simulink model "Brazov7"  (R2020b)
settings: Solver=VariableStepAuto  StartTime=0.0  StopTime=10.0  RelTol=1e-3
model workspace: external: MAT-File (data not in the file)
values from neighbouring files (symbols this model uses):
  q1 = 0    [angles.m]
  q2 = 90    [angles.m]
  q3 = 90    [angles.m]
  q4 = 0    [angles.m]
  q5 = 0    [angles.m]
undefined symbols (not defined in the file or in its folder): deg, kg, m, mm, N, s, smiData, X, Y, Z
libraries: sm_lib x30, nesl_utility x6

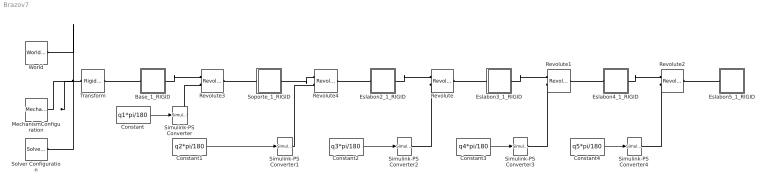
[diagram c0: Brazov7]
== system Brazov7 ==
  Base_1_RIGID : Subsystem
  Constant : Constant  Value=q1*pi/180
  Constant1 : Constant  Value=q2*pi/180
  Constant2 : Constant  Value=q3*pi/180
  Constant3 : Constant  Value=q4*pi/180
  Constant4 : Constant  Value=q5*pi/180
  Eslabon2_1_RIGID : Subsystem
  Eslabon3_1_RIGID : Subsystem
  Eslabon4_1_RIGID : Subsystem
  Eslabon5_1_RIGID : Subsystem
  MechanismConfiguration : sm_lib/Utilities/Mechanism Configuration  UniformGravity=Constant  GravityVector=[0 -9.80665 0]  GravityVectorUnits=m/s^2  GravityUnits=m/s^2  LinearizationDelta=0.001  JointModeTransitionNonlinearIterations=2
  Revolute : sm_lib/Joints/Revolute Joint  JointMode=Normal  SenseConstraintForce=off  SenseConstraintForceX=off  SenseConstraintForceY=off  SenseConstraintForceZ=off  SenseConstraintTorque=off  SenseConstraintTorqueX=off  SenseConstraintTorqueY=off  SenseConstraintTorqueZ=off  SenseTotalForce=off  SenseTotalForceX=off  SenseTotalForceY=off  SenseTotalForceZ=off  SenseTotalTorque=off  SenseTotalTorqueX=off  SenseTotalTorqueY=off  SenseTotalTorqueZ=off  CompositeWrenchDir=FollowerOnBase  CompositeWrenchFrame=BaseFrame  EquilibriumPosition=0  EquilibriumPositionUnits=deg  SpringStiffness=0  SpringStiffnessUnits=N*m/deg  DampingCoefficient=0  DampingCoefficientUnits=N*m/(deg/s)  TorqueActuationMode=ComputedTorque  MotionActuationMode=InputMotion  SensePosition=off  SenseVelocity=off  SenseAcceleration=off  SenseTorqueForce=off  SenseLowerLimitTorqueForce=off  SenseUpperLimitTorqueForce=off  LowerLimitSpecify=off  LowerLimitBound=-90  LowerLimitBoundUnits=deg  LowerLimitStiffness=1e4  LowerLimitStiffnessUnits=N*m/deg  LowerLimitDamping=10  LowerLimitDampingUnits=N*m/(deg/s)  LowerLimitTransitionRegionWidth=0.1  LowerLimitTransitionRegionWidthUnits=deg  UpperLimitSpecify=off  UpperLimitBound=90  UpperLimitBoundUnits=deg  UpperLimitStiffness=1e4  UpperLimitStiffnessUnits=N*m/deg  UpperLimitDamping=10  UpperLimitDampingUnits=N*m/(deg/s)  UpperLimitTransitionRegionWidth=0.1  UpperLimitTransitionRegionWidthUnits=deg  PositionTargetSpecify=on  PositionTargetPriority=Low  PositionTargetValue=smiData.RevoluteJoint(1).Rz.Pos  PositionTargetValueUnits=deg  VelocityTargetSpecify=off  VelocityTargetPriority=High  VelocityTargetValue=0  VelocityTargetValueUnits=deg/s
  Revolute1 : sm_lib/Joints/Revolute Joint  JointMode=Normal  SenseConstraintForce=off  SenseConstraintForceX=off  SenseConstraintForceY=off  SenseConstraintForceZ=off  SenseConstraintTorque=off  SenseConstraintTorqueX=off  SenseConstraintTorqueY=off  SenseConstraintTorqueZ=off  SenseTotalForce=off  SenseTotalForceX=off  SenseTotalForceY=off  SenseTotalForceZ=off  SenseTotalTorque=off  SenseTotalTorqueX=off  SenseTotalTorqueY=off  SenseTotalTorqueZ=off  CompositeWrenchDir=FollowerOnBase  CompositeWrenchFrame=BaseFrame  EquilibriumPosition=0  EquilibriumPositionUnits=deg  SpringStiffness=0  SpringStiffnessUnits=N*m/deg  DampingCoefficient=0  DampingCoefficientUnits=N*m/(deg/s)  TorqueActuationMode=ComputedTorque  MotionActuationMode=InputMotion  SensePosition=off  SenseVelocity=off  SenseAcceleration=off  SenseTorqueForce=off  SenseLowerLimitTorqueForce=off  SenseUpperLimitTorqueForce=off  LowerLimitSpecify=off  LowerLimitBound=-90  LowerLimitBoundUnits=deg  LowerLimitStiffness=1e4  LowerLimitStiffnessUnits=N*m/deg  LowerLimitDamping=10  LowerLimitDampingUnits=N*m/(deg/s)  LowerLimitTransitionRegionWidth=0.1  LowerLimitTransitionRegionWidthUnits=deg  UpperLimitSpecify=off  UpperLimitBound=90  UpperLimitBoundUnits=deg  UpperLimitStiffness=1e4  UpperLimitStiffnessUnits=N*m/deg  UpperLimitDamping=10  UpperLimitDampingUnits=N*m/(deg/s)  UpperLimitTransitionRegionWidth=0.1  UpperLimitTransitionRegionWidthUnits=deg  PositionTargetSpecify=on  PositionTargetPriority=Low  PositionTargetValue=smiData.RevoluteJoint(2).Rz.Pos  PositionTargetValueUnits=deg  VelocityTargetSpecify=off  VelocityTargetPriority=High  VelocityTargetValue=0  VelocityTargetValueUnits=deg/s
  Revolute2 : sm_lib/Joints/Revolute Joint  JointMode=Normal  SenseConstraintForce=off  SenseConstraintForceX=off  SenseConstraintForceY=off  SenseConstraintForceZ=off  SenseConstraintTorque=off  SenseConstraintTorqueX=off  SenseConstraintTorqueY=off  SenseConstraintTorqueZ=off  SenseTotalForce=off  SenseTotalForceX=off  SenseTotalForceY=off  SenseTotalForceZ=off  SenseTotalTorque=off  SenseTotalTorqueX=off  SenseTotalTorqueY=off  SenseTotalTorqueZ=off  CompositeWrenchDir=FollowerOnBase  CompositeWrenchFrame=BaseFrame  EquilibriumPosition=0  EquilibriumPositionUnits=deg  SpringStiffness=0  SpringStiffnessUnits=N*m/deg  DampingCoefficient=0  DampingCoefficientUnits=N*m/(deg/s)  TorqueActuationMode=ComputedTorque  MotionActuationMode=InputMotion  SensePosition=off  SenseVelocity=off  SenseAcceleration=off  SenseTorqueForce=off  SenseLowerLimitTorqueForce=off  SenseUpperLimitTorqueForce=off  LowerLimitSpecify=off  LowerLimitBound=-90  LowerLimitBoundUnits=deg  LowerLimitStiffness=1e4  LowerLimitStiffnessUnits=N*m/deg  LowerLimitDamping=10  LowerLimitDampingUnits=N*m/(deg/s)  LowerLimitTransitionRegionWidth=0.1  LowerLimitTransitionRegionWidthUnits=deg  UpperLimitSpecify=off  UpperLimitBound=90  UpperLimitBoundUnits=deg  UpperLimitStiffness=1e4  UpperLimitStiffnessUnits=N*m/deg  UpperLimitDamping=10  UpperLimitDampingUnits=N*m/(deg/s)  UpperLimitTransitionRegionWidth=0.1  UpperLimitTransitionRegionWidthUnits=deg  PositionTargetSpecify=on  PositionTargetPriority=Low  PositionTargetValue=smiData.RevoluteJoint(3).Rz.Pos  PositionTargetValueUnits=deg  VelocityTargetSpecify=off  VelocityTargetPriority=High  VelocityTargetValue=0  VelocityTargetValueUnits=deg/s
  Revolute3 : sm_lib/Joints/Revolute Joint  JointMode=Normal  SenseConstraintForce=off  SenseConstraintForceX=off  SenseConstraintForceY=off  SenseConstraintForceZ=off  SenseConstraintTorque=off  SenseConstraintTorqueX=off  SenseConstraintTorqueY=off  SenseConstraintTorqueZ=off  SenseTotalForce=off  SenseTotalForceX=off  SenseTotalForceY=off  SenseTotalForceZ=off  SenseTotalTorque=off  SenseTotalTorqueX=off  SenseTotalTorqueY=off  SenseTotalTorqueZ=off  CompositeWrenchDir=FollowerOnBase  CompositeWrenchFrame=BaseFrame  EquilibriumPosition=0  EquilibriumPositionUnits=deg  SpringStiffness=0  SpringStiffnessUnits=N*m/deg  DampingCoefficient=0  DampingCoefficientUnits=N*m/(deg/s)  TorqueActuationMode=ComputedTorque  MotionActuationMode=InputMotion  SensePosition=off  SenseVelocity=off  SenseAcceleration=off  SenseTorqueForce=off  SenseLowerLimitTorqueForce=off  SenseUpperLimitTorqueForce=off  LowerLimitSpecify=off  LowerLimitBound=-90  LowerLimitBoundUnits=deg  LowerLimitStiffness=1e4  LowerLimitStiffnessUnits=N*m/deg  LowerLimitDamping=10  LowerLimitDampingUnits=N*m/(deg/s)  LowerLimitTransitionRegionWidth=0.1  LowerLimitTransitionRegionWidthUnits=deg  UpperLimitSpecify=off  UpperLimitBound=90  UpperLimitBoundUnits=deg  UpperLimitStiffness=1e4  UpperLimitStiffnessUnits=N*m/deg  UpperLimitDamping=10  UpperLimitDampingUnits=N*m/(deg/s)  UpperLimitTransitionRegionWidth=0.1  UpperLimitTransitionRegionWidthUnits=deg  PositionTargetSpecify=on  PositionTargetPriority=Low  PositionTargetValue=smiData.RevoluteJoint(4).Rz.Pos  PositionTargetValueUnits=deg  VelocityTargetSpecify=off  VelocityTargetPriority=High  VelocityTargetValue=0  VelocityTargetValueUnits=deg/s
  Revolute4 : sm_lib/Joints/Revolute Joint  JointMode=Normal  SenseConstraintForce=off  SenseConstraintForceX=off  SenseConstraintForceY=off  SenseConstraintForceZ=off  SenseConstraintTorque=off  SenseConstraintTorqueX=off  SenseConstraintTorqueY=off  SenseConstraintTorqueZ=off  SenseTotalForce=off  SenseTotalForceX=off  SenseTotalForceY=off  SenseTotalForceZ=off  SenseTotalTorque=off  SenseTotalTorqueX=off  SenseTotalTorqueY=off  SenseTotalTorqueZ=off  CompositeWrenchDir=FollowerOnBase  CompositeWrenchFrame=BaseFrame  EquilibriumPosition=0  EquilibriumPositionUnits=deg  SpringStiffness=0  SpringStiffnessUnits=N*m/deg  DampingCoefficient=0  DampingCoefficientUnits=N*m/(deg/s)  TorqueActuationMode=ComputedTorque  MotionActuationMode=InputMotion  SensePosition=off  SenseVelocity=off  SenseAcceleration=off  SenseTorqueForce=off  SenseLowerLimitTorqueForce=off  SenseUpperLimitTorqueForce=off  LowerLimitSpecify=off  LowerLimitBound=-90  LowerLimitBoundUnits=deg  LowerLimitStiffness=1e4  LowerLimitStiffnessUnits=N*m/deg  LowerLimitDamping=10  LowerLimitDampingUnits=N*m/(deg/s)  LowerLimitTransitionRegionWidth=0.1  LowerLimitTransitionRegionWidthUnits=deg  UpperLimitSpecify=off  UpperLimitBound=90  UpperLimitBoundUnits=deg  UpperLimitStiffness=1e4  UpperLimitStiffnessUnits=N*m/deg  UpperLimitDamping=10  UpperLimitDampingUnits=N*m/(deg/s)  UpperLimitTransitionRegionWidth=0.1  UpperLimitTransitionRegionWidthUnits=deg  PositionTargetSpecify=on  PositionTargetPriority=Low  PositionTargetValue=smiData.RevoluteJoint(5).Rz.Pos  PositionTargetValueUnits=deg  VelocityTargetSpecify=off  VelocityTargetPriority=High  VelocityTargetValue=0  VelocityTargetValueUnits=deg/s
  Simulink-PS Converter{,1..4} (5 alike) : nesl_utility/Simulink-PS Converter  PhysicalDomain=network_engine_domain  SubClassName=ps_input  LeftPortType=input  RightPortType=output  PseudoPeriodic=off  Frequencies=[]  NoiseDistribution=none  NoiseParameters=[]  Unit=1  AffineConversion=off  FilteringAndDerivatives=filter  SimscapeFilterOrder=2  InputFilterTimeConstant=0.001  UdotUserProvided=0
  Solver Configuration : nesl_utility/Solver Configuration  PhysicalDomain=network_engine_domain  SubClassName=solver  LeftPortType=input  RightPortType=generic  Tones=[]  Harmonics=[]  SimulateNoise=off  Profile=off  UseLocalSampling=off  EnableSwitchedLinearOptims=on  FrequencyDomain=off  UseCCode=off  RelTol=0.001  AbsTol=1e-06  MinStep=1e-09  ToWorkspace=off  RevertToSquareIcSolve=off  NumHomotopyIterations=100  PhasorMode=off  PhasorModeNumHarmonics=1  DoDC=off  ResidualTolerance=1e-09  UseLocalSolver=off  LocalSolverChoice=NE_BACKWARD_EULER_ADVANCER  LocalSolverSampleTime=0.001  DoFixedCost=off  MaxNonlinIter=3  MaxModeIter=2  ComputeImpulses=off  ImpulseIterations=2  LinearAlgebra=auto  EquationFormulation=NE_TIME_EF  DelaysMemoryBudget=1024  AutomaticFiltering=on  FilteringTimeConstant=0.001  PartitionStorageMethod=AS_NEEDED  PartitionMemoryBudget=1024  PartitionMethod=ROBUST
  Soporte_1_RIGID : Subsystem
  Transform : sm_lib/Frames and Transforms/Rigid Transform  TranslationMethod=Cartesian  TranslationStandardOffset=0  TranslationLengthUnit=mm  TranslationStandardAxis=+Z  TranslationCartesianOffset=smiData.RigidTransform(11).translation  TranslationROffset=0  TranslationROffsetUnits=m  TranslationZOffset=0  TranslationZOffsetUnits=m  TranslationThetaOffset=0  TranslationThetaOffsetUnits=deg  RotationMethod=ArbitraryAxis  RotationAngleUnits=rad  RotationStandardAxis=+Z  RotationAngle=smiData.RigidTransform(11).angle  RotationArbitraryAxis=smiData.RigidTransform(11).axis  FollAlignAxisA=+X  BaseAlignAxisA=+Y  FollAlignAxisB=+Y  BaseAlignAxisB=+Z  RotationSequenceAxes=FollowerAxes  RotationSequence=XYX  RotationSequenceAngles=[0 0 0]  RotationSequenceAnglesUnits=deg  RotationMatrix=[1 0 0; 0 1 0; 0 0 1]
  World : sm_lib/Frames and Transforms/World Frame
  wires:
  Constant/1 -> Simulink-PS Converter/1
  Constant1/1 -> Simulink-PS Converter1/1
  Constant2/1 -> Simulink-PS Converter2/1
  Constant3/1 -> Simulink-PS Converter3/1
  Constant4/1 -> Simulink-PS Converter4/1
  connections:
  Transform/LConn1 -- MechanismConfiguration/RConn1 -- Solver Configuration/RConn1 -- World/RConn1
  Eslabon2_1_RIGID/RConn1 -- Revolute/LConn1
  Eslabon2_1_RIGID/LConn1 -- Revolute4/RConn1
  Base_1_RIGID/LConn1 -- Transform/RConn1
  Eslabon3_1_RIGID/LConn1 -- Revolute/RConn1
  Eslabon3_1_RIGID/RConn1 -- Revolute1/LConn1
  Eslabon4_1_RIGID/LConn1 -- Revolute1/RConn1
  Eslabon4_1_RIGID/RConn1 -- Revolute2/LConn1
  Eslabon5_1_RIGID/LConn1 -- Revolute2/RConn1
  Base_1_RIGID/RConn1 -- Revolute3/LConn1
  Revolute3/RConn1 -- Soporte_1_RIGID/LConn1
  Revolute4/LConn1 -- Soporte_1_RIGID/RConn1
  Simulink-PS Converter/RConn1 -- Revolute3/LConn2
  Simulink-PS Converter1/RConn1 -- Revolute4/LConn2
  Revolute/LConn2 -- Simulink-PS Converter2/RConn1
  Revolute1/LConn2 -- Simulink-PS Converter3/RConn1
  Revolute2/LConn2 -- Simulink-PS Converter4/RConn1

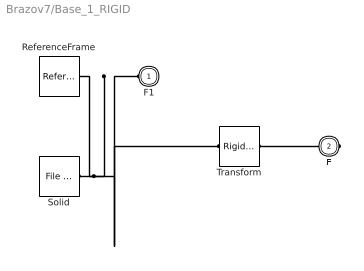
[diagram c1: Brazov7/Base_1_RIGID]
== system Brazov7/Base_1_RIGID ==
  ReferenceFrame : sm_lib/Frames and Transforms/Reference Frame
  Solid : sm_lib/Body Elements/File Solid  ExtGeomFileName=Base_Default_sldprt.STEP  UnitType=FromFile  ExtGeomFileUnits=m  StepReaderType=HEX  ExportConvexHullGeometry=off  InertiaType=Custom  Mass=smiData.Solid(1).mass  MassUnits=kg  CenterOfMass=smiData.Solid(1).CoM  CenterOfMassUnits=mm  MomentsOfInertia=smiData.Solid(1).MoI  MomentsOfInertiaUnits=kg*mm^2  ProductsOfInertia=smiData.Solid(1).PoI  ProductsOfInertiaUnits=kg*mm^2  BasedOnType=DensityFromFile  Density=1000  DensityUnits=kg/m^3  DoExposeReferenceFrame=on  SerializedFrames=<Frames/>  GraphicType=FromGeometry  MarkerShape=Sphere  MarkerSize=10  GraphicVisPropType=SimpleVisualProperties  GraphicDiffuseColor=smiData.Solid(1).color  GraphicSpecularColor=[0.5 0.5 0.5 1.0]  GraphicAmbientColor=[0.15 0.15 0.15 1.0]  GraphicEmissiveColor=[0.0 0.0 0.0 1.0]  GraphicShininess=75  GraphicOpacity=smiData.Solid(1).opacity
  Transform : sm_lib/Frames and Transforms/Rigid Transform  TranslationMethod=Cartesian  TranslationStandardOffset=0  TranslationLengthUnit=mm  TranslationStandardAxis=+Z  TranslationCartesianOffset=smiData.RigidTransform(7).translation  TranslationROffset=0  TranslationROffsetUnits=m  TranslationZOffset=0  TranslationZOffsetUnits=m  TranslationThetaOffset=0  TranslationThetaOffsetUnits=deg  RotationMethod=ArbitraryAxis  RotationAngleUnits=rad  RotationStandardAxis=+Z  RotationAngle=smiData.RigidTransform(7).angle  RotationArbitraryAxis=smiData.RigidTransform(7).axis  FollAlignAxisA=+X  BaseAlignAxisA=+Y  FollAlignAxisB=+Y  BaseAlignAxisB=+Z  RotationSequenceAxes=FollowerAxes  RotationSequence=XYX  RotationSequenceAngles=[0 0 0]  RotationSequenceAnglesUnits=deg  RotationMatrix=[1 0 0; 0 1 0; 0 0 1]
  F1 : PMIOPort  Side=Left
  F : PMIOPort  Port=2  Side=Right
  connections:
  Solid/RConn1 -- ReferenceFrame/RConn1 -- Transform/LConn1 -- F1/RConn1
  Transform/RConn1 -- F/RConn1

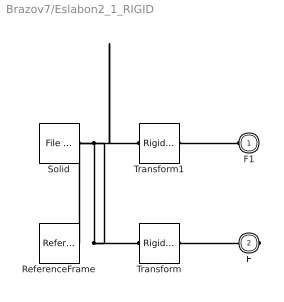
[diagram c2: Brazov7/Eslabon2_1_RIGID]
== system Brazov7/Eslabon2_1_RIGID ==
  ReferenceFrame : sm_lib/Frames and Transforms/Reference Frame
  Solid : sm_lib/Body Elements/File Solid  ExtGeomFileName=Eslabon2_Default_sldprt.STEP  UnitType=FromFile  ExtGeomFileUnits=m  StepReaderType=HEX  ExportConvexHullGeometry=off  InertiaType=Custom  Mass=smiData.Solid(3).mass  MassUnits=kg  CenterOfMass=smiData.Solid(3).CoM  CenterOfMassUnits=mm  MomentsOfInertia=smiData.Solid(3).MoI  MomentsOfInertiaUnits=kg*mm^2  ProductsOfInertia=smiData.Solid(3).PoI  ProductsOfInertiaUnits=kg*mm^2  BasedOnType=DensityFromFile  Density=1000  DensityUnits=kg/m^3  DoExposeReferenceFrame=on  SerializedFrames=<Frames/>  GraphicType=FromGeometry  MarkerShape=Sphere  MarkerSize=10  GraphicVisPropType=SimpleVisualProperties  GraphicDiffuseColor=smiData.Solid(3).color  GraphicSpecularColor=[0.5 0.5 0.5 1.0]  GraphicAmbientColor=[0.15 0.15 0.15 1.0]  GraphicEmissiveColor=[0.0 0.0 0.0 1.0]  GraphicShininess=75  GraphicOpacity=smiData.Solid(3).opacity
  Transform : sm_lib/Frames and Transforms/Rigid Transform  TranslationMethod=Cartesian  TranslationStandardOffset=0  TranslationLengthUnit=mm  TranslationStandardAxis=+Z  TranslationCartesianOffset=smiData.RigidTransform(1).translation  TranslationROffset=0  TranslationROffsetUnits=m  TranslationZOffset=0  TranslationZOffsetUnits=m  TranslationThetaOffset=0  TranslationThetaOffsetUnits=deg  RotationMethod=ArbitraryAxis  RotationAngleUnits=rad  RotationStandardAxis=+Z  RotationAngle=smiData.RigidTransform(1).angle  RotationArbitraryAxis=smiData.RigidTransform(1).axis  FollAlignAxisA=+X  BaseAlignAxisA=+Y  FollAlignAxisB=+Y  BaseAlignAxisB=+Z  RotationSequenceAxes=FollowerAxes  RotationSequence=XYX  RotationSequenceAngles=[0 0 0]  RotationSequenceAnglesUnits=deg  RotationMatrix=[1 0 0; 0 1 0; 0 0 1]
  Transform1 : sm_lib/Frames and Transforms/Rigid Transform  TranslationMethod=Cartesian  TranslationStandardOffset=0  TranslationLengthUnit=mm  TranslationStandardAxis=+Z  TranslationCartesianOffset=smiData.RigidTransform(10).translation  TranslationROffset=0  TranslationROffsetUnits=m  TranslationZOffset=0  TranslationZOffsetUnits=m  TranslationThetaOffset=0  TranslationThetaOffsetUnits=deg  RotationMethod=ArbitraryAxis  RotationAngleUnits=rad  RotationStandardAxis=+Z  RotationAngle=smiData.RigidTransform(10).angle  RotationArbitraryAxis=smiData.RigidTransform(10).axis  FollAlignAxisA=+X  BaseAlignAxisA=+Y  FollAlignAxisB=+Y  BaseAlignAxisB=+Z  RotationSequenceAxes=FollowerAxes  RotationSequence=XYX  RotationSequenceAngles=[0 0 0]  RotationSequenceAnglesUnits=deg  RotationMatrix=[1 0 0; 0 1 0; 0 0 1]
  F1 : PMIOPort  Side=Left
  F : PMIOPort  Port=2  Side=Right
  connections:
  Solid/RConn1 -- ReferenceFrame/RConn1 -- Transform/LConn1 -- Transform1/LConn1
  Transform/RConn1 -- F/RConn1
  Transform1/RConn1 -- F1/RConn1

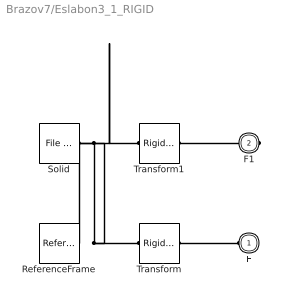
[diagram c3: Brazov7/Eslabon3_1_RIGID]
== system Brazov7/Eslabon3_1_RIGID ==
  ReferenceFrame : sm_lib/Frames and Transforms/Reference Frame
  Solid : sm_lib/Body Elements/File Solid  ExtGeomFileName=Eslabon3_Default_sldprt.STEP  UnitType=FromFile  ExtGeomFileUnits=m  StepReaderType=HEX  ExportConvexHullGeometry=off  InertiaType=Custom  Mass=smiData.Solid(4).mass  MassUnits=kg  CenterOfMass=smiData.Solid(4).CoM  CenterOfMassUnits=mm  MomentsOfInertia=smiData.Solid(4).MoI  MomentsOfInertiaUnits=kg*mm^2  ProductsOfInertia=smiData.Solid(4).PoI  ProductsOfInertiaUnits=kg*mm^2  BasedOnType=DensityFromFile  Density=1000  DensityUnits=kg/m^3  DoExposeReferenceFrame=on  SerializedFrames=<Frames/>  GraphicType=FromGeometry  MarkerShape=Sphere  MarkerSize=10  GraphicVisPropType=SimpleVisualProperties  GraphicDiffuseColor=smiData.Solid(4).color  GraphicSpecularColor=[0.5 0.5 0.5 1.0]  GraphicAmbientColor=[0.15 0.15 0.15 1.0]  GraphicEmissiveColor=[0.0 0.0 0.0 1.0]  GraphicShininess=75  GraphicOpacity=smiData.Solid(4).opacity
  Transform : sm_lib/Frames and Transforms/Rigid Transform  TranslationMethod=Cartesian  TranslationStandardOffset=0  TranslationLengthUnit=mm  TranslationStandardAxis=+Z  TranslationCartesianOffset=smiData.RigidTransform(2).translation  TranslationROffset=0  TranslationROffsetUnits=m  TranslationZOffset=0  TranslationZOffsetUnits=m  TranslationThetaOffset=0  TranslationThetaOffsetUnits=deg  RotationMethod=ArbitraryAxis  RotationAngleUnits=rad  RotationStandardAxis=+Z  RotationAngle=smiData.RigidTransform(2).angle  RotationArbitraryAxis=smiData.RigidTransform(2).axis  FollAlignAxisA=+X  BaseAlignAxisA=+Y  FollAlignAxisB=+Y  BaseAlignAxisB=+Z  RotationSequenceAxes=FollowerAxes  RotationSequence=XYX  RotationSequenceAngles=[0 0 0]  RotationSequenceAnglesUnits=deg  RotationMatrix=[1 0 0; 0 1 0; 0 0 1]
  Transform1 : sm_lib/Frames and Transforms/Rigid Transform  TranslationMethod=Cartesian  TranslationStandardOffset=0  TranslationLengthUnit=mm  TranslationStandardAxis=+Z  TranslationCartesianOffset=smiData.RigidTransform(3).translation  TranslationROffset=0  TranslationROffsetUnits=m  TranslationZOffset=0  TranslationZOffsetUnits=m  TranslationThetaOffset=0  TranslationThetaOffsetUnits=deg  RotationMethod=ArbitraryAxis  RotationAngleUnits=rad  RotationStandardAxis=+Z  RotationAngle=smiData.RigidTransform(3).angle  RotationArbitraryAxis=smiData.RigidTransform(3).axis  FollAlignAxisA=+X  BaseAlignAxisA=+Y  FollAlignAxisB=+Y  BaseAlignAxisB=+Z  RotationSequenceAxes=FollowerAxes  RotationSequence=XYX  RotationSequenceAngles=[0 0 0]  RotationSequenceAnglesUnits=deg  RotationMatrix=[1 0 0; 0 1 0; 0 0 1]
  F : PMIOPort  Side=Left
  F1 : PMIOPort  Port=2  Side=Right
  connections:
  Solid/RConn1 -- ReferenceFrame/RConn1 -- Transform/LConn1 -- Transform1/LConn1
  Transform/RConn1 -- F/RConn1
  Transform1/RConn1 -- F1/RConn1

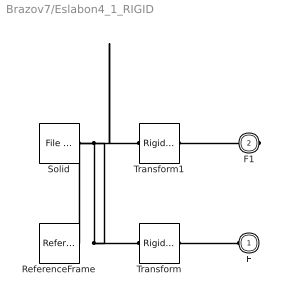
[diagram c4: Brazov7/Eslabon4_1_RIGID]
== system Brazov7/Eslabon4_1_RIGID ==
  ReferenceFrame : sm_lib/Frames and Transforms/Reference Frame
  Solid : sm_lib/Body Elements/File Solid  ExtGeomFileName=Eslabon4_Default_sldprt.STEP  UnitType=FromFile  ExtGeomFileUnits=m  StepReaderType=HEX  ExportConvexHullGeometry=off  InertiaType=Custom  Mass=smiData.Solid(6).mass  MassUnits=kg  CenterOfMass=smiData.Solid(6).CoM  CenterOfMassUnits=mm  MomentsOfInertia=smiData.Solid(6).MoI  MomentsOfInertiaUnits=kg*mm^2  ProductsOfInertia=smiData.Solid(6).PoI  ProductsOfInertiaUnits=kg*mm^2  BasedOnType=DensityFromFile  Density=1000  DensityUnits=kg/m^3  DoExposeReferenceFrame=on  SerializedFrames=<Frames/>  GraphicType=FromGeometry  MarkerShape=Sphere  MarkerSize=10  GraphicVisPropType=SimpleVisualProperties  GraphicDiffuseColor=smiData.Solid(6).color  GraphicSpecularColor=[0.5 0.5 0.5 1.0]  GraphicAmbientColor=[0.15 0.15 0.15 1.0]  GraphicEmissiveColor=[0.0 0.0 0.0 1.0]  GraphicShininess=75  GraphicOpacity=smiData.Solid(6).opacity
  Transform : sm_lib/Frames and Transforms/Rigid Transform  TranslationMethod=Cartesian  TranslationStandardOffset=0  TranslationLengthUnit=mm  TranslationStandardAxis=+Z  TranslationCartesianOffset=smiData.RigidTransform(4).translation  TranslationROffset=0  TranslationROffsetUnits=m  TranslationZOffset=0  TranslationZOffsetUnits=m  TranslationThetaOffset=0  TranslationThetaOffsetUnits=deg  RotationMethod=ArbitraryAxis  RotationAngleUnits=rad  RotationStandardAxis=+Z  RotationAngle=smiData.RigidTransform(4).angle  RotationArbitraryAxis=smiData.RigidTransform(4).axis  FollAlignAxisA=+X  BaseAlignAxisA=+Y  FollAlignAxisB=+Y  BaseAlignAxisB=+Z  RotationSequenceAxes=FollowerAxes  RotationSequence=XYX  RotationSequenceAngles=[0 0 0]  RotationSequenceAnglesUnits=deg  RotationMatrix=[1 0 0; 0 1 0; 0 0 1]
  Transform1 : sm_lib/Frames and Transforms/Rigid Transform  TranslationMethod=Cartesian  TranslationStandardOffset=0  TranslationLengthUnit=mm  TranslationStandardAxis=+Z  TranslationCartesianOffset=smiData.RigidTransform(5).translation  TranslationROffset=0  TranslationROffsetUnits=m  TranslationZOffset=0  TranslationZOffsetUnits=m  TranslationThetaOffset=0  TranslationThetaOffsetUnits=deg  RotationMethod=ArbitraryAxis  RotationAngleUnits=rad  RotationStandardAxis=+Z  RotationAngle=smiData.RigidTransform(5).angle  RotationArbitraryAxis=smiData.RigidTransform(5).axis  FollAlignAxisA=+X  BaseAlignAxisA=+Y  FollAlignAxisB=+Y  BaseAlignAxisB=+Z  RotationSequenceAxes=FollowerAxes  RotationSequence=XYX  RotationSequenceAngles=[0 0 0]  RotationSequenceAnglesUnits=deg  RotationMatrix=[1 0 0; 0 1 0; 0 0 1]
  F : PMIOPort  Side=Left
  F1 : PMIOPort  Port=2  Side=Right
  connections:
  Solid/RConn1 -- ReferenceFrame/RConn1 -- Transform/LConn1 -- Transform1/LConn1
  Transform/RConn1 -- F/RConn1
  Transform1/RConn1 -- F1/RConn1

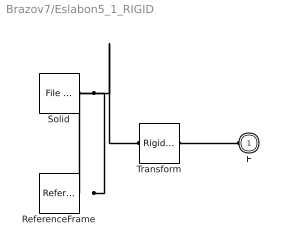
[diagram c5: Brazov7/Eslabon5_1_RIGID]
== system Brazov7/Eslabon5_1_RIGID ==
  ReferenceFrame : sm_lib/Frames and Transforms/Reference Frame
  Solid : sm_lib/Body Elements/File Solid  ExtGeomFileName=Eslabon5_Default_sldprt.STEP  UnitType=FromFile  ExtGeomFileUnits=m  StepReaderType=HEX  ExportConvexHullGeometry=off  InertiaType=Custom  Mass=smiData.Solid(5).mass  MassUnits=kg  CenterOfMass=smiData.Solid(5).CoM  CenterOfMassUnits=mm  MomentsOfInertia=smiData.Solid(5).MoI  MomentsOfInertiaUnits=kg*mm^2  ProductsOfInertia=smiData.Solid(5).PoI  ProductsOfInertiaUnits=kg*mm^2  BasedOnType=DensityFromFile  Density=1000  DensityUnits=kg/m^3  DoExposeReferenceFrame=on  SerializedFrames=<Frames/>  GraphicType=FromGeometry  MarkerShape=Sphere  MarkerSize=10  GraphicVisPropType=SimpleVisualProperties  GraphicDiffuseColor=smiData.Solid(5).color  GraphicSpecularColor=[0.5 0.5 0.5 1.0]  GraphicAmbientColor=[0.15 0.15 0.15 1.0]  GraphicEmissiveColor=[0.0 0.0 0.0 1.0]  GraphicShininess=75  GraphicOpacity=smiData.Solid(5).opacity
  Transform : sm_lib/Frames and Transforms/Rigid Transform  TranslationMethod=Cartesian  TranslationStandardOffset=0  TranslationLengthUnit=mm  TranslationStandardAxis=+Z  TranslationCartesianOffset=smiData.RigidTransform(6).translation  TranslationROffset=0  TranslationROffsetUnits=m  TranslationZOffset=0  TranslationZOffsetUnits=m  TranslationThetaOffset=0  TranslationThetaOffsetUnits=deg  RotationMethod=ArbitraryAxis  RotationAngleUnits=rad  RotationStandardAxis=+Z  RotationAngle=smiData.RigidTransform(6).angle  RotationArbitraryAxis=smiData.RigidTransform(6).axis  FollAlignAxisA=+X  BaseAlignAxisA=+Y  FollAlignAxisB=+Y  BaseAlignAxisB=+Z  RotationSequenceAxes=FollowerAxes  RotationSequence=XYX  RotationSequenceAngles=[0 0 0]  RotationSequenceAnglesUnits=deg  RotationMatrix=[1 0 0; 0 1 0; 0 0 1]
  F : PMIOPort  Side=Left
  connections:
  Solid/RConn1 -- ReferenceFrame/RConn1 -- Transform/LConn1
  Transform/RConn1 -- F/RConn1

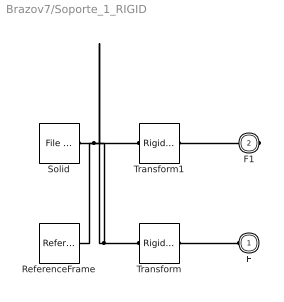
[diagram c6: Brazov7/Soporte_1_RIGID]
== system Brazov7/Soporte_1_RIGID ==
  ReferenceFrame : sm_lib/Frames and Transforms/Reference Frame
  Solid : sm_lib/Body Elements/File Solid  ExtGeomFileName=Soporte_Default_sldprt.STEP  UnitType=FromFile  ExtGeomFileUnits=m  StepReaderType=HEX  ExportConvexHullGeometry=off  InertiaType=Custom  Mass=smiData.Solid(2).mass  MassUnits=kg  CenterOfMass=smiData.Solid(2).CoM  CenterOfMassUnits=mm  MomentsOfInertia=smiData.Solid(2).MoI  MomentsOfInertiaUnits=kg*mm^2  ProductsOfInertia=smiData.Solid(2).PoI  ProductsOfInertiaUnits=kg*mm^2  BasedOnType=DensityFromFile  Density=1000  DensityUnits=kg/m^3  DoExposeReferenceFrame=on  SerializedFrames=<Frames/>  GraphicType=FromGeometry  MarkerShape=Sphere  MarkerSize=10  GraphicVisPropType=SimpleVisualProperties  GraphicDiffuseColor=smiData.Solid(2).color  GraphicSpecularColor=[0.5 0.5 0.5 1.0]  GraphicAmbientColor=[0.15 0.15 0.15 1.0]  GraphicEmissiveColor=[0.0 0.0 0.0 1.0]  GraphicShininess=75  GraphicOpacity=smiData.Solid(2).opacity
  Transform : sm_lib/Frames and Transforms/Rigid Transform  TranslationMethod=Cartesian  TranslationStandardOffset=0  TranslationLengthUnit=mm  TranslationStandardAxis=+Z  TranslationCartesianOffset=smiData.RigidTransform(8).translation  TranslationROffset=0  TranslationROffsetUnits=m  TranslationZOffset=0  TranslationZOffsetUnits=m  TranslationThetaOffset=0  TranslationThetaOffsetUnits=deg  RotationMethod=ArbitraryAxis  RotationAngleUnits=rad  RotationStandardAxis=+Z  RotationAngle=smiData.RigidTransform(8).angle  RotationArbitraryAxis=smiData.RigidTransform(8).axis  FollAlignAxisA=+X  BaseAlignAxisA=+Y  FollAlignAxisB=+Y  BaseAlignAxisB=+Z  RotationSequenceAxes=FollowerAxes  RotationSequence=XYX  RotationSequenceAngles=[0 0 0]  RotationSequenceAnglesUnits=deg  RotationMatrix=[1 0 0; 0 1 0; 0 0 1]
  Transform1 : sm_lib/Frames and Transforms/Rigid Transform  TranslationMethod=Cartesian  TranslationStandardOffset=0  TranslationLengthUnit=mm  TranslationStandardAxis=+Z  TranslationCartesianOffset=smiData.RigidTransform(9).translation  TranslationROffset=0  TranslationROffsetUnits=m  TranslationZOffset=0  TranslationZOffsetUnits=m  TranslationThetaOffset=0  TranslationThetaOffsetUnits=deg  RotationMethod=ArbitraryAxis  RotationAngleUnits=rad  RotationStandardAxis=+Z  RotationAngle=smiData.RigidTransform(9).angle  RotationArbitraryAxis=smiData.RigidTransform(9).axis  FollAlignAxisA=+X  BaseAlignAxisA=+Y  FollAlignAxisB=+Y  BaseAlignAxisB=+Z  RotationSequenceAxes=FollowerAxes  RotationSequence=XYX  RotationSequenceAngles=[0 0 0]  RotationSequenceAnglesUnits=deg  RotationMatrix=[1 0 0; 0 1 0; 0 0 1]
  F : PMIOPort  Side=Left
  F1 : PMIOPort  Port=2  Side=Right
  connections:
  Solid/RConn1 -- ReferenceFrame/RConn1 -- Transform/LConn1 -- Transform1/LConn1
  Transform/RConn1 -- F/RConn1
  Transform1/RConn1 -- F1/RConn1
